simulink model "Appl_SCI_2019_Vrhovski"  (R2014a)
settings: Solver=ode45  StartTime=0.0  StopTime=1000  MaxStep=0.01  RelTol=1e-3
undefined symbols (not defined in the file): deg, H, kg, m, M, mm, N, rad, s, X, Y, Z
libraries: sm_lib x389, nesl_utility x69, simulink x7
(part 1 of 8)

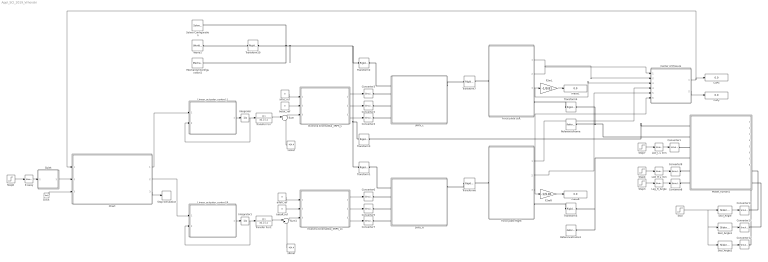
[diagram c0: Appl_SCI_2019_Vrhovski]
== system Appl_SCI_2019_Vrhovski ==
  3RPS_L : Subsystem
  3RPS_R : Subsystem
  Center of Presure : MATLAB Function  TreatAsAtomicUnit=on
  Chart : Stateflow chart  TreatAsAtomicUnit=on
  Clock : Clock
  CoPx : Display
  CoPy : Display
  Converter{1..7,9} (8 alike) : nesl_utility/Simulink-PS Converter  PhysicalDomain=network_engine_domain  SubClassName=ps_input  LeftPortType=input  RightPortType=output  PseudoPeriodic=off  Frequencies=[]  NoiseDistribution=none  NoiseParameters=[]  Unit=mm  AffineConversion=off  InputFiltering=on  SimscapeFilterOrder=2  InputFilterTimeConstant=.01  UdotUserProvided=1
  Converter{8,10..12} (4 alike) : nesl_utility/Simulink-PS Converter  PhysicalDomain=network_engine_domain  SubClassName=ps_input  LeftPortType=input  RightPortType=output  PseudoPeriodic=off  Frequencies=[]  NoiseDistribution=none  NoiseParameters=[]  Unit=rad  AffineConversion=off  InputFiltering=on  SimscapeFilterOrder=2  InputFilterTimeConstant=.01  UdotUserProvided=1
  F2mL : Gain  Gain=-1/9.81
  F2mR : Gain  Gain=-1/9.81
  Force plate Left : Subsystem
  Force plate Right : Subsystem
  Integrator : Integrator
  Integrator1 : Integrator
  Inverzna kinematika_3RPS_L : MATLAB Function  TreatAsAtomicUnit=on
  Inverzna kinematika_3RPS_L1 : MATLAB Function  TreatAsAtomicUnit=on
  K sway : simulink/Math Operations/Slider Gain  low=0  gain=0  high=1
  LLD_L u mm : simulink/Math Operations/Slider Gain  low=0  gain=25  high=340
  LLD_R u mm : simulink/Math Operations/Slider Gain  low=0  gain=0  high=100
  Leg_R_Angle : simulink/Math Operations/Slider Gain  low=-1  gain=0  high=30
  Linear_actuator_control_L : MATLAB Function  TreatAsAtomicUnit=on
  Linear_actuator_control_R : MATLAB Function  TreatAsAtomicUnit=on
  MechanismConfiguration1 : sm_lib/Utilities/Mechanism Configuration  UniformGravity=Constant  GravityVector="[0  0 -9.81]"  GravityUnits=m/s^2  LinearizationDelta=0.001  BlockFunction=simmechanics.library.utilities.mechanism_configuration
  Model_human1 : Subsystem
  Quiet : MATLAB Function  TreatAsAtomicUnit=on
  ReferenceFrame : sm_lib/Frames and Transforms/Reference Frame  BlockFunction=simmechanics.library.frames_transforms.reference_frame
  ReferenceFrame1 : sm_lib/Frames and Transforms/Reference Frame  BlockFunction=simmechanics.library.frames_transforms.reference_frame
  Skol : Step  Time=0  SampleTime=0
  Skol_Angle : simulink/Math Operations/Slider Gain  low=-1  gain=-0.192  high=1
  Skol_Angle1 : simulink/Math Operations/Slider Gain  low=-2  gain=0.078199  high=1
  Skol_Angle2 : simulink/Math Operations/Slider Gain  low=-1  gain=0.09701  high=1
  Solver Configuration : nesl_utility/Solver Configuration  PhysicalDomain=network_engine_domain  SubClassName=solver  LeftPortType=input  RightPortType=generic  Accelerate=off  Tones=[]  Harmonics=[]  SimulateNoise=off  Profile=off  UseLocalSampling=off  EnableSwitchedLinearOptims=on  FrequencyDomain=off  UseCCode=off  RelTol=0.001  AbsTol=1e-06  MinStep=1e-09  ToWorkspace=off  DoDC=off  ResidualTolerance=1e-06  UseLocalSolver=off  LocalSolverChoice=NE_BACKWARD_EULER_ADVANCER  LocalSolverSampleTime=0.001  DoFixedCost=off  MaxNonlinIter=3  MaxModeIter=2  LinearAlgebra=Sparse  DelaysMemoryBudget=1024  AutomaticFiltering=on  FilteringTimeConstant=0.001
  Step3 : Step  Time=0  After=-1  SampleTime=0
  Step4 : Step  Time=0  SampleTime=0
  Step6 : Step  Time=0  SampleTime=0
  Step7 : Step  Time=0  SampleTime=0
  Stop Simulation : Stop
  Sum : Sum  Inputs=|++
  Sum1 : Sum  Inputs=|++
  Transfer Fcn : TransferFcn  Denominator=[0.3 1]
  Transfer Fcn1 : TransferFcn  Denominator=[0.3 1]
  Transform1 : sm_lib/Frames and Transforms/Rigid Transform  TranslationMethod=Cartesian  TranslationLengthUnit=mm  TranslationStandardAxis=+Z  TranslationStandardOffset=0  TranslationCartesianOffset=[0 265 2.5]  TranslationROffset=0  TranslationROffsetUnits=m  TranslationZOffset=0  TranslationZOffsetUnits=m  TranslationThetaOffset=0  TranslationThetaOffsetUnits=deg  RotationMethod=None  RotationAngleUnits=rad  RotationStandardAxis=+Z  RotationAngle=0.66591007177581396  RotationArbitraryAxis=[0.82933268280998906 0.55820538845577061 0.024779941931496435]  FollAlignAxisA=+X  BaseAlignAxisA=+Y  FollAlignAxisB=+Y  BaseAlignAxisB=+Z  BlockFunction=simmechanics.library.frames_transforms.rigid_transform
  Transform10 : sm_lib/Frames and Transforms/Rigid Transform  TranslationMethod=None  TranslationLengthUnit=mm  TranslationStandardAxis=+Z  TranslationStandardOffset=2.5  TranslationCartesianOffset=[0 0 0]  TranslationROffset=0  TranslationROffsetUnits=m  TranslationZOffset=0  TranslationZOffsetUnits=m  TranslationThetaOffset=0  TranslationThetaOffsetUnits=deg  RotationMethod=StandardAxis  RotationAngleUnits=rad  RotationStandardAxis=-Z  RotationAngle=pi/2  RotationArbitraryAxis=[0.82933268280998906 0.55820538845577061 0.024779941931496435]  FollAlignAxisA=+X  BaseAlignAxisA=+Y  FollAlignAxisB=+Y  BaseAlignAxisB=+Z  BlockFunction=simmechanics.library.frames_transforms.rigid_transform
  Transform2 : sm_lib/Frames and Transforms/Rigid Transform  TranslationMethod=Cartesian  TranslationLengthUnit=mm  TranslationStandardAxis=+Z  TranslationStandardOffset=2.5  TranslationCartesianOffset=[0 0 2.5]  TranslationROffset=0  TranslationROffsetUnits=m  TranslationZOffset=0  TranslationZOffsetUnits=m  TranslationThetaOffset=0  TranslationThetaOffsetUnits=deg  RotationMethod=None  RotationAngleUnits=rad  RotationStandardAxis=+Z  RotationAngle=0.66591007177581396  RotationArbitraryAxis=[0.82933268280998906 0.55820538845577061 0.024779941931496435]  FollAlignAxisA=+X  BaseAlignAxisA=+Y  FollAlignAxisB=+Y  BaseAlignAxisB=+Z  BlockFunction=simmechanics.library.frames_transforms.rigid_transform
  Transform3 : sm_lib/Frames and Transforms/Rigid Transform  TranslationMethod=Cartesian  TranslationLengthUnit=mm  TranslationStandardAxis=+Z  TranslationStandardOffset=2.5  TranslationCartesianOffset=[0 265/2 2.5]  TranslationROffset=0  TranslationROffsetUnits=m  TranslationZOffset=0  TranslationZOffsetUnits=m  TranslationThetaOffset=0  TranslationThetaOffsetUnits=deg  RotationMethod=None  RotationAngleUnits=rad  RotationStandardAxis=+Z  RotationAngle=0.66591007177581396  RotationArbitraryAxis=[0.82933268280998906 0.55820538845577061 0.024779941931496435]  FollAlignAxisA=+X  BaseAlignAxisA=+Y  FollAlignAxisB=+Y  BaseAlignAxisB=+Z  BlockFunction=simmechanics.library.frames_transforms.rigid_transform
  Transform4 : sm_lib/Frames and Transforms/Rigid Transform  TranslationMethod=Cartesian  TranslationLengthUnit=mm  TranslationStandardAxis=+Z  TranslationStandardOffset=15  TranslationCartesianOffset=[ 0 0 20]  TranslationROffset=0  TranslationROffsetUnits=m  TranslationZOffset=0  TranslationZOffsetUnits=m  TranslationThetaOffset=0  TranslationThetaOffsetUnits=deg  RotationMethod=None  RotationAngleUnits=rad  RotationStandardAxis=+Z  RotationAngle=2.0943951023931953  RotationArbitraryAxis=[-0.57735026918962584 -0.57735026918962584 -0.57735026918962584]  FollAlignAxisA=+X  BaseAlignAxisA=+Y  FollAlignAxisB=+Y  BaseAlignAxisB=+Z  BlockFunction=simmechanics.library.frames_transforms.rigid_transform
  Transform5 : sm_lib/Frames and Transforms/Rigid Transform  TranslationMethod=Cartesian  TranslationLengthUnit=mm  TranslationStandardAxis=+Z  TranslationStandardOffset=15  TranslationCartesianOffset=[ 0 0 20]  TranslationROffset=0  TranslationROffsetUnits=m  TranslationZOffset=0  TranslationZOffsetUnits=m  TranslationThetaOffset=0  TranslationThetaOffsetUnits=deg  RotationMethod=None  RotationAngleUnits=rad  RotationStandardAxis=+Z  RotationAngle=2.0943951023931953  RotationArbitraryAxis=[-0.57735026918962584 -0.57735026918962584 -0.57735026918962584]  FollAlignAxisA=+X  BaseAlignAxisA=+Y  FollAlignAxisB=+Y  BaseAlignAxisB=+Z  BlockFunction=simmechanics.library.frames_transforms.rigid_transform
  Transform6 : sm_lib/Frames and Transforms/Rigid Transform  TranslationMethod=None  TranslationLengthUnit=mm  TranslationStandardAxis=+Z  TranslationStandardOffset=54.83  TranslationCartesianOffset=[-120 50 70]  TranslationROffset=0  TranslationROffsetUnits=m  TranslationZOffset=0  TranslationZOffsetUnits=m  TranslationThetaOffset=0  TranslationThetaOffsetUnits=deg  RotationMethod=StandardAxis  RotationAngleUnits=rad  RotationStandardAxis=+Z  RotationAngle=pi/2  RotationArbitraryAxis=[0 0 0]  FollAlignAxisA=+X  BaseAlignAxisA=+Y  FollAlignAxisB=+Y  BaseAlignAxisB=+Z  BlockFunction=simmechanics.library.frames_transforms.rigid_transform
  Transform7 : sm_lib/Frames and Transforms/Rigid Transform  TranslationMethod=None  TranslationLengthUnit=mm  TranslationStandardAxis=+Z  TranslationStandardOffset=54.83  TranslationCartesianOffset=[-120 50 70]  TranslationROffset=0  TranslationROffsetUnits=m  TranslationZOffset=0  TranslationZOffsetUnits=m  TranslationThetaOffset=0  TranslationThetaOffsetUnits=deg  RotationMethod=StandardAxis  RotationAngleUnits=rad  RotationStandardAxis=+Z  RotationAngle=pi/2  RotationArbitraryAxis=[0 0 0]  FollAlignAxisA=+X  BaseAlignAxisA=+Y  FollAlignAxisB=+Y  BaseAlignAxisB=+Z  BlockFunction=simmechanics.library.frames_transforms.rigid_transform
  World1 : sm_lib/Frames and Transforms/World Frame  BlockFunction=simmechanics.library.frames_transforms.world_frame
  alfaL_ref : Constant  Value=0
  alfaR_ref : Constant  Value=0
  betaL_ref : Constant  Value=0
  betaR_ref : Constant  Value=0
  masaL : Display
  masaR : Display
  zL0ref : Constant  Value=424.4
  zR0ref : Constant  Value=424.4
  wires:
  Force plate Left/1(CoP_x) -> Center of Presure/1(CoPxL)
  Force plate Left/2(CoP_y) -> Center of Presure/2(CoPyL)
  Force plate Right/1(CoP_x) -> Center of Presure/4(CoPxR)
  Force plate Right/2(CoP_y) -> Center of Presure/5(CoPyR)
  Step7/1 -> LLD_L u mm/1
  LLD_L u mm/1 -> Converter1/1
  Step3/1 -> Leg_R_Angle/1
  Step4/1 -> LLD_R u mm/1
  LLD_R u mm/1 -> Converter9/1
  Force plate Right/3(Fz) -> F2mR/1, Center of Presure/6(FzR)
  F2mL/1 -> masaL/1
  F2mR/1 -> masaR/1
  Force plate Left/3(Fz) -> F2mL/1, Center of Presure/3(FzL)
  Center of Presure/2(CoP_y) -> CoPy/1
  Leg_R_Angle/1 -> Converter8/1
  Inverzna kinematika_3RPS_L/1(d1) -> Converter3/1
  Inverzna kinematika_3RPS_L/2(d2) -> Converter2/1
  Inverzna kinematika_3RPS_L/3(d3) -> Converter4/1
  Inverzna kinematika_3RPS_L1/1(d1) -> Converter6/1
  Inverzna kinematika_3RPS_L1/2(d2) -> Converter5/1
  Inverzna kinematika_3RPS_L1/3(d3) -> Converter7/1
  Center of Presure/1(CoP_x) -> Chart/1(CoM_x), CoPx/1
  alfaL_ref/1 -> Inverzna kinematika_3RPS_L/1(alfa)
  betaL_ref/1 -> Inverzna kinematika_3RPS_L/2(beta)
  alfaR_ref/1 -> Inverzna kinematika_3RPS_L1/1(alfa)
  betaR_ref/1 -> Inverzna kinematika_3RPS_L1/2(beta)
  zL0ref/1 -> Sum/2
  Transfer Fcn1/1 -> Sum1/1
  Sum1/1 -> Inverzna kinematika_3RPS_L1/3(z)
  zR0ref/1 -> Sum1/2
  Skol/1 -> Skol_Angle2/1, Skol_Angle1/1, Skol_Angle/1
  Linear_actuator_control_L/1(u_R) -> Integrator/1
  Integrator/1 -> Linear_actuator_control_L/2(delta_z), Transfer Fcn/1
  Transfer Fcn/1 -> Sum/1
  Linear_actuator_control_R/1(u_R) -> Integrator1/1
  Integrator1/1 -> Transfer Fcn1/1, Linear_actuator_control_R/2(delta_z)
  K sway/1 -> Quiet/1(u)
  Step6/1 -> K sway/1
  Clock/1 -> Chart/3(t)
  Chart/3(end_sim) -> Stop Simulation/1
  Quiet/1(y) -> Chart/2(Q)
  Chart/1(z_ref_L) -> Linear_actuator_control_L/1(delta_z_ref)
  Chart/2(z_ref_R) -> Linear_actuator_control_R/1(delta_z_ref)
  Sum/1 -> Inverzna kinematika_3RPS_L/3(z)
  Skol_Angle2/1 -> Converter12/1
  Skol_Angle1/1 -> Converter11/1
  Skol_Angle/1 -> Converter10/1
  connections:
  3RPS_L/LConn1 -- Transform2/RConn1
  3RPS_L/RConn1 -- Transform7/LConn1
  3RPS_R/LConn1 -- Transform1/RConn1
  Transform6/LConn1 -- 3RPS_R/RConn1
  Transform4/RConn1 -- Model_human1/LConn2 -- ReferenceFrame/RConn1
  Transform5/RConn1 -- Model_human1/LConn4 -- ReferenceFrame1/RConn1
  Model_human1/LConn5 -- Converter9/RConn1
  Transform4/LConn1 -- Force plate Left/RConn1
  Transform5/LConn1 -- Force plate Right/RConn1
  Model_human1/LConn3 -- Converter1/RConn1
  Model_human1/LConn6 -- Converter8/RConn1
  Transform10/RConn1 -- Solver Configuration/RConn1 -- MechanismConfiguration1/RConn1 -- Transform1/LConn1 -- Transform3/LConn1 -- Transform2/LConn1
  Transform7/RConn1 -- Force plate Left/LConn1
  Transform6/RConn1 -- Force plate Right/LConn1
  Transform10/LConn1 -- World1/RConn1
  3RPS_R/LConn4 -- Converter7/RConn1
  3RPS_R/LConn3 -- Converter5/RConn1
  3RPS_R/LConn2 -- Converter6/RConn1
  3RPS_L/LConn2 -- Converter3/RConn1
  3RPS_L/LConn3 -- Converter2/RConn1
  3RPS_L/LConn4 -- Converter4/RConn1
  Transform3/RConn1 -- Model_human1/LConn1
  Model_human1/RConn1 -- Converter10/RConn1
  Model_human1/RConn3 -- Converter11/RConn1
  Converter12/RConn1 -- Model_human1/RConn2

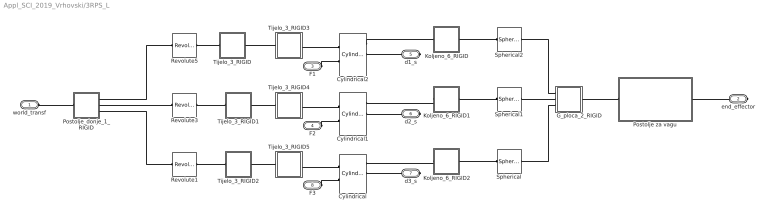
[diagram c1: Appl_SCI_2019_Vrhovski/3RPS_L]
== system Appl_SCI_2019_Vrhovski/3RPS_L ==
  Cylindrical : sm_lib/Joints/Cylindrical Joint  SenseConstraintForce=off  SenseConstraintForceX=off  SenseConstraintForceY=off  SenseConstraintForceZ=off  SenseConstraintTorque=off  SenseConstraintTorqueX=off  SenseConstraintTorqueY=off  SenseConstraintTorqueZ=off  SenseTotalForce=off  SenseTotalForceX=off  SenseTotalForceY=off  SenseTotalForceZ=off  SenseTotalTorque=off  SenseTotalTorqueX=off  SenseTotalTorqueY=off  SenseTotalTorqueZ=off  CompositeWrenchDir=FollowerOnBase  CompositeWrenchFrame=BaseFrame  PzEquilibriumPosition=0  PzEquilibriumPositionUnits=m  PzSpringStiffness=0  PzSpringStiffnessUnits=N/m  PzDampingCoefficient=0  PzDampingCoefficientUnits=s*N/m  PzTorqueActuationMode=ComputedTorque  PzMotionActuationMode=InputMotion  PzSensePosition=on  PzSenseVelocity=on  PzSenseAcceleration=off  PzSenseTorqueForce=off  PzPositionTargetValue=0  PzPositionTargetValueUnits=mm  PzPositionTargetSpecify=on  PzPositionTargetPriority=Low  PzVelocityTargetValue=0  PzVelocityTargetValueUnits=m/s  PzVelocityTargetSpecify=off  PzVelocityTargetPriority=High  RzEquilibriumPosition=0  RzEquilibriumPositionUnits=rad  RzSpringStiffness=0  RzSpringStiffnessUnits=m*N/rad  RzDampingCoefficient=0  RzDampingCoefficientUnits=m*s*N/rad  RzTorqueActuationMode=NoTorque  RzMotionActuationMode=ComputedMotion  RzSensePosition=off  RzSenseVelocity=off  RzSenseAcceleration=off  RzSenseTorqueForce=off  RzPositionTargetValue=149.99999999999969  RzPositionTargetValueUnits=deg  RzPositionTargetSpecify=on  RzPositionTargetPriority=Low  RzVelocityTargetValue=0  RzVelocityTargetValueUnits=deg/s  RzVelocityTargetSpecify=off  RzVelocityTargetPriority=High  BlockFunction=simmechanics.library.joints.cylindrical_joint
  Cylindrical1 : sm_lib/Joints/Cylindrical Joint  SenseConstraintForce=off  SenseConstraintForceX=off  SenseConstraintForceY=off  SenseConstraintForceZ=off  SenseConstraintTorque=off  SenseConstraintTorqueX=off  SenseConstraintTorqueY=off  SenseConstraintTorqueZ=off  SenseTotalForce=off  SenseTotalForceX=off  SenseTotalForceY=off  SenseTotalForceZ=off  SenseTotalTorque=off  SenseTotalTorqueX=off  SenseTotalTorqueY=off  SenseTotalTorqueZ=off  CompositeWrenchDir=FollowerOnBase  CompositeWrenchFrame=BaseFrame  PzEquilibriumPosition=0  PzEquilibriumPositionUnits=m  PzSpringStiffness=0  PzSpringStiffnessUnits=N/m  PzDampingCoefficient=0  PzDampingCoefficientUnits=s*N/m  PzTorqueActuationMode=ComputedTorque  PzMotionActuationMode=InputMotion  PzSensePosition=on  PzSenseVelocity=on  PzSenseAcceleration=off  PzSenseTorqueForce=off  PzPositionTargetValue=0  PzPositionTargetValueUnits=mm  PzPositionTargetSpecify=on  PzPositionTargetPriority=High  PzVelocityTargetValue=0  PzVelocityTargetValueUnits=m/s  PzVelocityTargetSpecify=off  PzVelocityTargetPriority=High  RzEquilibriumPosition=0  RzEquilibriumPositionUnits=rad  RzSpringStiffness=0  RzSpringStiffnessUnits=m*N/rad  RzDampingCoefficient=0  RzDampingCoefficientUnits=m*s*N/rad  RzTorqueActuationMode=NoTorque  RzMotionActuationMode=ComputedMotion  RzSensePosition=off  RzSenseVelocity=off  RzSenseAcceleration=off  RzSenseTorqueForce=off  RzPositionTargetValue=1.1114762716872906  RzPositionTargetValueUnits=deg  RzPositionTargetSpecify=on  RzPositionTargetPriority=Low  RzVelocityTargetValue=0  RzVelocityTargetValueUnits=deg/s  RzVelocityTargetSpecify=off  RzVelocityTargetPriority=High  BlockFunction=simmechanics.library.joints.cylindrical_joint
  Cylindrical2 : sm_lib/Joints/Cylindrical Joint  SenseConstraintForce=off  SenseConstraintForceX=off  SenseConstraintForceY=off  SenseConstraintForceZ=off  SenseConstraintTorque=off  SenseConstraintTorqueX=off  SenseConstraintTorqueY=off  SenseConstraintTorqueZ=off  SenseTotalForce=off  SenseTotalForceX=off  SenseTotalForceY=off  SenseTotalForceZ=off  SenseTotalTorque=off  SenseTotalTorqueX=off  SenseTotalTorqueY=off  SenseTotalTorqueZ=off  CompositeWrenchDir=FollowerOnBase  CompositeWrenchFrame=BaseFrame  PzEquilibriumPosition=0  PzEquilibriumPositionUnits=m  PzSpringStiffness=0  PzSpringStiffnessUnits=N/m  PzDampingCoefficient=0  PzDampingCoefficientUnits=s*N/m  PzTorqueActuationMode=ComputedTorque  PzMotionActuationMode=InputMotion  PzSensePosition=on  PzSenseVelocity=on  PzSenseAcceleration=off  PzSenseTorqueForce=off  PzPositionTargetValue=0  PzPositionTargetValueUnits=mm  PzPositionTargetSpecify=on  PzPositionTargetPriority=High  PzVelocityTargetValue=0  PzVelocityTargetValueUnits=m/s  PzVelocityTargetSpecify=off  PzVelocityTargetPriority=High  RzEquilibriumPosition=0  RzEquilibriumPositionUnits=rad  RzSpringStiffness=0  RzSpringStiffnessUnits=m*N/rad  RzDampingCoefficient=0  RzDampingCoefficientUnits=m*s*N/rad  RzTorqueActuationMode=NoTorque  RzMotionActuationMode=ComputedMotion  RzSensePosition=off  RzSenseVelocity=off  RzSenseAcceleration=off  RzSenseTorqueForce=off  RzPositionTargetValue=-128.14822527507599  RzPositionTargetValueUnits=deg  RzPositionTargetSpecify=on  RzPositionTargetPriority=Low  RzVelocityTargetValue=0  RzVelocityTargetValueUnits=deg/s  RzVelocityTargetSpecify=off  RzVelocityTargetPriority=High  BlockFunction=simmechanics.library.joints.cylindrical_joint
  G_ploca_2_RIGID : Subsystem
  Koljeno_6_RIGID : Subsystem
  Koljeno_6_RIGID1 : Subsystem
  Koljeno_6_RIGID2 : Subsystem
  Postolje za vagu : Subsystem
  Postolje_donje_1_RIGID : Subsystem
  Revolute1 : sm_lib/Joints/Revolute Joint  SenseConstraintForce=off  SenseConstraintForceX=off  SenseConstraintForceY=off  SenseConstraintForceZ=off  SenseConstraintTorque=off  SenseConstraintTorqueX=off  SenseConstraintTorqueY=off  SenseConstraintTorqueZ=off  SenseTotalForce=off  SenseTotalForceX=off  SenseTotalForceY=off  SenseTotalForceZ=off  SenseTotalTorque=off  SenseTotalTorqueX=off  SenseTotalTorqueY=off  SenseTotalTorqueZ=off  CompositeWrenchDir=FollowerOnBase  CompositeWrenchFrame=BaseFrame  EquilibriumPosition=0  EquilibriumPositionUnits=rad  SpringStiffness=0  SpringStiffnessUnits=m*N/rad  DampingCoefficient=0  DampingCoefficientUnits=m*s*N/rad  TorqueActuationMode=NoTorque  MotionActuationMode=ComputedMotion  SensePosition=off  SenseVelocity=off  SenseAcceleration=off  SenseTorqueForce=off  PositionTargetValue=-169.15902616998602  PositionTargetValueUnits=deg  PositionTargetSpecify=on  PositionTargetPriority=Low  VelocityTargetValue=0  VelocityTargetValueUnits=deg/s  VelocityTargetSpecify=off  VelocityTargetPriority=High  BlockFunction=simmechanics.library.joints.revolute_joint
  Revolute3 : sm_lib/Joints/Revolute Joint  SenseConstraintForce=off  SenseConstraintForceX=off  SenseConstraintForceY=off  SenseConstraintForceZ=off  SenseConstraintTorque=off  SenseConstraintTorqueX=off  SenseConstraintTorqueY=off  SenseConstraintTorqueZ=off  SenseTotalForce=off  SenseTotalForceX=off  SenseTotalForceY=off  SenseTotalForceZ=off  SenseTotalTorque=off  SenseTotalTorqueX=off  SenseTotalTorqueY=off  SenseTotalTorqueZ=off  CompositeWrenchDir=FollowerOnBase  CompositeWrenchFrame=BaseFrame  EquilibriumPosition=0  EquilibriumPositionUnits=rad  SpringStiffness=0  SpringStiffnessUnits=m*N/rad  DampingCoefficient=0  DampingCoefficientUnits=m*s*N/rad  TorqueActuationMode=NoTorque  MotionActuationMode=ComputedMotion  SensePosition=off  SenseVelocity=off  SenseAcceleration=off  SenseTorqueForce=off  PositionTargetValue=169.15902616998767  PositionTargetValueUnits=deg  PositionTargetSpecify=on  PositionTargetPriority=Low  VelocityTargetValue=0  VelocityTargetValueUnits=deg/s  VelocityTargetSpecify=off  VelocityTargetPriority=High  BlockFunction=simmechanics.library.joints.revolute_joint
  Revolute5 : sm_lib/Joints/Revolute Joint  SenseConstraintForce=off  SenseConstraintForceX=off  SenseConstraintForceY=off  SenseConstraintForceZ=off  SenseConstraintTorque=off  SenseConstraintTorqueX=off  SenseConstraintTorqueY=off  SenseConstraintTorqueZ=off  SenseTotalForce=off  SenseTotalForceX=off  SenseTotalForceY=off  SenseTotalForceZ=off  SenseTotalTorque=off  SenseTotalTorqueX=off  SenseTotalTorqueY=off  SenseTotalTorqueZ=off  CompositeWrenchDir=FollowerOnBase  CompositeWrenchFrame=BaseFrame  EquilibriumPosition=0  EquilibriumPositionUnits=rad  SpringStiffness=0  SpringStiffnessUnits=m*N/rad  DampingCoefficient=0  DampingCoefficientUnits=m*s*N/rad  TorqueActuationMode=NoTorque  MotionActuationMode=ComputedMotion  SensePosition=off  SenseVelocity=off  SenseAcceleration=off  SenseTorqueForce=off  PositionTargetValue=79.159026169986646  PositionTargetValueUnits=deg  PositionTargetSpecify=on  PositionTargetPriority=Low  VelocityTargetValue=0  VelocityTargetValueUnits=deg/s  VelocityTargetSpecify=off  VelocityTargetPriority=High  BlockFunction=simmechanics.library.joints.revolute_joint
  Spherical : sm_lib/Joints/Spherical Joint  SenseConstraintForce=off  SenseConstraintForceX=off  SenseConstraintForceY=off  SenseConstraintForceZ=off  SenseConstraintTorque=off  SenseConstraintTorqueX=off  SenseConstraintTorqueY=off  SenseConstraintTorqueZ=off  SenseTotalForce=off  SenseTotalForceX=off  SenseTotalForceY=off  SenseTotalForceZ=off  SenseTotalTorque=off  SenseTotalTorqueX=off  SenseTotalTorqueY=off  SenseTotalTorqueZ=off  CompositeWrenchDir=FollowerOnBase  CompositeWrenchFrame=BaseFrame  DefPosRotationMethod=None  DefPosRotationAngleUnits=deg  DefPosRotationStandardAxis=+Z  DefPosRotationAngle=0  DefPosRotationArbitraryAxis=[0 0 1]  DefPosFollAlignAxisA=+X  DefPosBaseAlignAxisA=+Y  DefPosFollAlignAxisB=+Y  DefPosBaseAlignAxisB=+Z  EqPosRotationMethod=None  EqPosRotationAngleUnits=deg  EqPosRotationStandardAxis=+Z  EqPosRotationAngle=0  EqPosRotationArbitraryAxis=[0 0 1]  EqPosFollAlignAxisA=+X  EqPosBaseAlignAxisA=+Y  EqPosFollAlignAxisB=+Y  EqPosBaseAlignAxisB=+Z  SpringStiffness=0  SpringStiffnessUnits=m*N/rad  DampingCoefficient=0  DampingCoefficientUnits=m*s*N/rad  ActuateTorqueX=off  ActuateTorqueY=off  ActuateTorqueZ=off  ActuateTorque=off  TorqueActuationMode=NoTorque  MotionActuationMode=ComputedMotion  ActuationFrame=BaseFrame  SensePosition=off  SenseVelocityX=off  SenseVelocityY=off  SenseVelocityZ=off  SenseVelocity=off  SenseAccelerationX=off  SenseAccelerationY=off  SenseAccelerationZ=off  SenseAcceleration=off  SenseTorqueX=off  SenseTorqueY=off  SenseTorqueZ=off  SenseTorqueForce=off  SensingFrame=FollowerFrame  PositionTargetRotationMethod=ArbitraryAxis  PositionTargetRotationAngleUnits=deg  PositionTargetRotationStandardAxis=+Z  PositionTargetRotationAngle=99.696739951188775  PositionTargetRotationArbitraryAxis=[-0.99752584719718795 0.068907511443980704 -0.013926199773456341]  PositionTargetFollAlignAxisA=+X  PositionTargetBaseAlignAxisA=+Y  PositionTargetFollAlignAxisB=+Y  PositionTargetBaseAlignAxisB=+Z  PositionTargetSpecify=on  PositionTargetPriority=Low  VelocityTargetValue=[0 0 0]  VelocityTargetValueUnits=deg/s  VelocityTargetSpecify=off  VelocityTargetPriority=High  VelocityTargetInFollowerFrame=on  BlockFunction=simmechanics.library.joints.spherical_joint
  Spherical1 : sm_lib/Joints/Spherical Joint  SenseConstraintForce=off  SenseConstraintForceX=off  SenseConstraintForceY=off  SenseConstraintForceZ=off  SenseConstraintTorque=off  SenseConstraintTorqueX=off  SenseConstraintTorqueY=off  SenseConstraintTorqueZ=off  SenseTotalForce=off  SenseTotalForceX=off  SenseTotalForceY=off  SenseTotalForceZ=off  SenseTotalTorque=off  SenseTotalTorqueX=off  SenseTotalTorqueY=off  SenseTotalTorqueZ=off  CompositeWrenchDir=FollowerOnBase  CompositeWrenchFrame=BaseFrame  DefPosRotationMethod=None  DefPosRotationAngleUnits=deg  DefPosRotationStandardAxis=+Z  DefPosRotationAngle=0  DefPosRotationArbitraryAxis=[0 0 1]  DefPosFollAlignAxisA=+X  DefPosBaseAlignAxisA=+Y  DefPosFollAlignAxisB=+Y  DefPosBaseAlignAxisB=+Z  EqPosRotationMethod=None  EqPosRotationAngleUnits=deg  EqPosRotationStandardAxis=+Z  EqPosRotationAngle=0  EqPosRotationArbitraryAxis=[0 0 1]  EqPosFollAlignAxisA=+X  EqPosBaseAlignAxisA=+Y  EqPosFollAlignAxisB=+Y  EqPosBaseAlignAxisB=+Z  SpringStiffness=0  SpringStiffnessUnits=m*N/rad  DampingCoefficient=0  DampingCoefficientUnits=m*s*N/rad  ActuateTorqueX=off  ActuateTorqueY=off  ActuateTorqueZ=off  ActuateTorque=off  TorqueActuationMode=NoTorque  MotionActuationMode=ComputedMotion  ActuationFrame=BaseFrame  SensePosition=off  SenseVelocityX=off  SenseVelocityY=off  SenseVelocityZ=off  SenseVelocity=off  SenseAccelerationX=off  SenseAccelerationY=off  SenseAccelerationZ=off  SenseAcceleration=off  SenseTorqueX=off  SenseTorqueY=off  SenseTorqueZ=off  SenseTorqueForce=off  SensingFrame=FollowerFrame  PositionTargetRotationMethod=None  PositionTargetRotationAngleUnits=deg  PositionTargetRotationStandardAxis=+Z  PositionTargetRotationAngle=0  PositionTargetRotationArbitraryAxis=[0 0 1]  PositionTargetFollAlignAxisA=+X  PositionTargetBaseAlignAxisA=+Y  PositionTargetFollAlignAxisB=+Y  PositionTargetBaseAlignAxisB=+Z  PositionTargetSpecify=off  PositionTargetPriority=High  VelocityTargetValue=[0 0 0]  VelocityTargetValueUnits=deg/s  VelocityTargetSpecify=off  VelocityTargetPriority=High  VelocityTargetInFollowerFrame=on  BlockFunction=simmechanics.library.joints.spherical_joint
  Spherical2 : sm_lib/Joints/Spherical Joint  SenseConstraintForce=off  SenseConstraintForceX=off  SenseConstraintForceY=off  SenseConstraintForceZ=off  SenseConstraintTorque=off  SenseConstraintTorqueX=off  SenseConstraintTorqueY=off  SenseConstraintTorqueZ=off  SenseTotalForce=off  SenseTotalForceX=off  SenseTotalForceY=off  SenseTotalForceZ=off  SenseTotalTorque=off  SenseTotalTorqueX=off  SenseTotalTorqueY=off  SenseTotalTorqueZ=off  CompositeWrenchDir=FollowerOnBase  CompositeWrenchFrame=BaseFrame  DefPosRotationMethod=None  DefPosRotationAngleUnits=deg  DefPosRotationStandardAxis=+Z  DefPosRotationAngle=0  DefPosRotationArbitraryAxis=[0 0 1]  DefPosFollAlignAxisA=+X  DefPosBaseAlignAxisA=+Y  DefPosFollAlignAxisB=+Y  DefPosBaseAlignAxisB=+Z  EqPosRotationMethod=None  EqPosRotationAngleUnits=deg  EqPosRotationStandardAxis=+Z  EqPosRotationAngle=0  EqPosRotationArbitraryAxis=[0 0 1]  EqPosFollAlignAxisA=+X  EqPosBaseAlignAxisA=+Y  EqPosFollAlignAxisB=+Y  EqPosBaseAlignAxisB=+Z  SpringStiffness=0  SpringStiffnessUnits=m*N/rad  DampingCoefficient=0  DampingCoefficientUnits=m*s*N/rad  ActuateTorqueX=off  ActuateTorqueY=off  ActuateTorqueZ=off  ActuateTorque=off  TorqueActuationMode=NoTorque  MotionActuationMode=ComputedMotion  ActuationFrame=BaseFrame  SensePosition=off  SenseVelocityX=off  SenseVelocityY=off  SenseVelocityZ=off  SenseVelocity=off  SenseAccelerationX=off  SenseAccelerationY=off  SenseAccelerationZ=off  SenseAcceleration=off  SenseTorqueX=off  SenseTorqueY=off  SenseTorqueZ=off  SenseTorqueForce=off  SensingFrame=FollowerFrame  PositionTargetRotationMethod=None  PositionTargetRotationAngleUnits=deg  PositionTargetRotationStandardAxis=+Z  PositionTargetRotationAngle=0  PositionTargetRotationArbitraryAxis=[0 0 1]  PositionTargetFollAlignAxisA=+X  PositionTargetBaseAlignAxisA=+Y  PositionTargetFollAlignAxisB=+Y  PositionTargetBaseAlignAxisB=+Z  PositionTargetSpecify=off  PositionTargetPriority=High  VelocityTargetValue=[0 0 0]  VelocityTargetValueUnits=deg/s  VelocityTargetSpecify=off  VelocityTargetPriority=High  VelocityTargetInFollowerFrame=on  BlockFunction=simmechanics.library.joints.spherical_joint
  Tijelo_3_RIGID : Subsystem
  Tijelo_3_RIGID1 : Subsystem
  Tijelo_3_RIGID2 : Subsystem
  Tijelo_3_RIGID3 : Subsystem
  Tijelo_3_RIGID4 : Subsystem
  Tijelo_3_RIGID5 : Subsystem
  world_transf : PMIOPort  Port=1  Side=Left
  end_effector : PMIOPort  Port=2  Side=Right
  F1 : PMIOPort  Port=3  Side=Left
  F2 : PMIOPort  Port=4  Side=Left
  d1_s : PMIOPort  Port=5  Side=Right
  d2_s : PMIOPort  Port=6  Side=Right
  d3_s : PMIOPort  Port=7  Side=Right
  F3 : PMIOPort  Port=8  Side=Left
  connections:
  Postolje_donje_1_RIGID/RConn3 -- Revolute1/LConn1
  Koljeno_6_RIGID2/RConn1 -- Spherical/LConn1
  Koljeno_6_RIGID1/RConn1 -- Spherical1/LConn1
  G_ploca_2_RIGID/LConn2 -- Spherical1/RConn1
  G_ploca_2_RIGID/LConn1 -- Spherical2/RConn1
  G_ploca_2_RIGID/LConn3 -- Spherical/RConn1
  Revolute5/RConn1 -- Tijelo_3_RIGID/LConn1
  Koljeno_6_RIGID/RConn1 -- Spherical2/LConn1
  Postolje_donje_1_RIGID/RConn1 -- Revolute5/LConn1
  Tijelo_3_RIGID2/LConn1 -- Revolute1/RConn1
  Postolje_donje_1_RIGID/RConn2 -- Revolute3/LConn1
  d2_s/RConn1 -- Cylindrical1/RConn2
  d3_s/RConn1 -- Cylindrical/RConn2
  Cylindrical2/RConn1 -- Koljeno_6_RIGID/LConn1
  F3/RConn1 -- Cylindrical/LConn2
  d1_s/RConn1 -- Cylindrical2/RConn2
  Tijelo_3_RIGID1/LConn1 -- Revolute3/RConn1
  F1/RConn1 -- Cylindrical2/LConn2
  Koljeno_6_RIGID1/LConn1 -- Cylindrical1/RConn1
  F2/RConn1 -- Cylindrical1/LConn2
  Koljeno_6_RIGID2/LConn1 -- Cylindrical/RConn1
  world_transf/RConn1 -- Postolje_donje_1_RIGID/LConn1
  G_ploca_2_RIGID/RConn1 -- Postolje za vagu/LConn1
  Postolje za vagu/RConn1 -- end_effector/RConn1
  Tijelo_3_RIGID/RConn1 -- Tijelo_3_RIGID3/LConn1
  Tijelo_3_RIGID3/RConn1 -- Cylindrical2/LConn1
  Tijelo_3_RIGID1/RConn1 -- Tijelo_3_RIGID4/LConn1
  Tijelo_3_RIGID4/RConn1 -- Cylindrical1/LConn1
  Tijelo_3_RIGID2/RConn1 -- Tijelo_3_RIGID5/LConn1
  Tijelo_3_RIGID5/RConn1 -- Cylindrical/LConn1

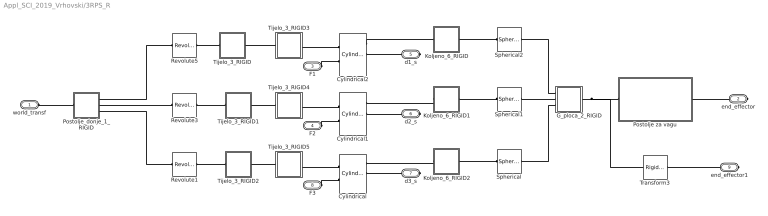
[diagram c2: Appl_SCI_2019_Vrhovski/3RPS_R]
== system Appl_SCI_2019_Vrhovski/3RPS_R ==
  Cylindrical : sm_lib/Joints/Cylindrical Joint  SenseConstraintForce=off  SenseConstraintForceX=off  SenseConstraintForceY=off  SenseConstraintForceZ=off  SenseConstraintTorque=off  SenseConstraintTorqueX=off  SenseConstraintTorqueY=off  SenseConstraintTorqueZ=off  SenseTotalForce=off  SenseTotalForceX=off  SenseTotalForceY=off  SenseTotalForceZ=off  SenseTotalTorque=off  SenseTotalTorqueX=off  SenseTotalTorqueY=off  SenseTotalTorqueZ=off  CompositeWrenchDir=FollowerOnBase  CompositeWrenchFrame=BaseFrame  PzEquilibriumPosition=0  PzEquilibriumPositionUnits=m  PzSpringStiffness=0  PzSpringStiffnessUnits=N/m  PzDampingCoefficient=0  PzDampingCoefficientUnits=s*N/m  PzTorqueActuationMode=ComputedTorque  PzMotionActuationMode=InputMotion  PzSensePosition=on  PzSenseVelocity=on  PzSenseAcceleration=off  PzSenseTorqueForce=off  PzPositionTargetValue=0  PzPositionTargetValueUnits=mm  PzPositionTargetSpecify=on  PzPositionTargetPriority=Low  PzVelocityTargetValue=0  PzVelocityTargetValueUnits=m/s  PzVelocityTargetSpecify=off  PzVelocityTargetPriority=High  RzEquilibriumPosition=0  RzEquilibriumPositionUnits=rad  RzSpringStiffness=0  RzSpringStiffnessUnits=m*N/rad  RzDampingCoefficient=0  RzDampingCoefficientUnits=m*s*N/rad  RzTorqueActuationMode=NoTorque  RzMotionActuationMode=ComputedMotion  RzSensePosition=off  RzSenseVelocity=off  RzSenseAcceleration=off  RzSenseTorqueForce=off  RzPositionTargetValue=149.99999999999969  RzPositionTargetValueUnits=deg  RzPositionTargetSpecify=on  RzPositionTargetPriority=Low  RzVelocityTargetValue=0  RzVelocityTargetValueUnits=deg/s  RzVelocityTargetSpecify=off  RzVelocityTargetPriority=High  BlockFunction=simmechanics.library.joints.cylindrical_joint
  Cylindrical1 : sm_lib/Joints/Cylindrical Joint  SenseConstraintForce=off  SenseConstraintForceX=off  SenseConstraintForceY=off  SenseConstraintForceZ=off  SenseConstraintTorque=off  SenseConstraintTorqueX=off  SenseConstraintTorqueY=off  SenseConstraintTorqueZ=off  SenseTotalForce=off  SenseTotalForceX=off  SenseTotalForceY=off  SenseTotalForceZ=off  SenseTotalTorque=off  SenseTotalTorqueX=off  SenseTotalTorqueY=off  SenseTotalTorqueZ=off  CompositeWrenchDir=FollowerOnBase  CompositeWrenchFrame=BaseFrame  PzEquilibriumPosition=0  PzEquilibriumPositionUnits=m  PzSpringStiffness=0  PzSpringStiffnessUnits=N/m  PzDampingCoefficient=0  PzDampingCoefficientUnits=s*N/m  PzTorqueActuationMode=ComputedTorque  PzMotionActuationMode=InputMotion  PzSensePosition=on  PzSenseVelocity=on  PzSenseAcceleration=off  PzSenseTorqueForce=off  PzPositionTargetValue=0  PzPositionTargetValueUnits=mm  PzPositionTargetSpecify=on  PzPositionTargetPriority=High  PzVelocityTargetValue=0  PzVelocityTargetValueUnits=m/s  PzVelocityTargetSpecify=off  PzVelocityTargetPriority=High  RzEquilibriumPosition=0  RzEquilibriumPositionUnits=rad  RzSpringStiffness=0  RzSpringStiffnessUnits=m*N/rad  RzDampingCoefficient=0  RzDampingCoefficientUnits=m*s*N/rad  RzTorqueActuationMode=NoTorque  RzMotionActuationMode=ComputedMotion  RzSensePosition=off  RzSenseVelocity=off  RzSenseAcceleration=off  RzSenseTorqueForce=off  RzPositionTargetValue=1.1114762716872906  RzPositionTargetValueUnits=deg  RzPositionTargetSpecify=on  RzPositionTargetPriority=Low  RzVelocityTargetValue=0  RzVelocityTargetValueUnits=deg/s  RzVelocityTargetSpecify=off  RzVelocityTargetPriority=High  BlockFunction=simmechanics.library.joints.cylindrical_joint
  Cylindrical2 : sm_lib/Joints/Cylindrical Joint  SenseConstraintForce=off  SenseConstraintForceX=off  SenseConstraintForceY=off  SenseConstraintForceZ=off  SenseConstraintTorque=off  SenseConstraintTorqueX=off  SenseConstraintTorqueY=off  SenseConstraintTorqueZ=off  SenseTotalForce=off  SenseTotalForceX=off  SenseTotalForceY=off  SenseTotalForceZ=off  SenseTotalTorque=off  SenseTotalTorqueX=off  SenseTotalTorqueY=off  SenseTotalTorqueZ=off  CompositeWrenchDir=FollowerOnBase  CompositeWrenchFrame=BaseFrame  PzEquilibriumPosition=0  PzEquilibriumPositionUnits=m  PzSpringStiffness=0  PzSpringStiffnessUnits=N/m  PzDampingCoefficient=0  PzDampingCoefficientUnits=s*N/m  PzTorqueActuationMode=ComputedTorque  PzMotionActuationMode=InputMotion  PzSensePosition=on  PzSenseVelocity=on  PzSenseAcceleration=off  PzSenseTorqueForce=off  PzPositionTargetValue=0  PzPositionTargetValueUnits=mm  PzPositionTargetSpecify=on  PzPositionTargetPriority=High  PzVelocityTargetValue=0  PzVelocityTargetValueUnits=m/s  PzVelocityTargetSpecify=off  PzVelocityTargetPriority=High  RzEquilibriumPosition=0  RzEquilibriumPositionUnits=rad  RzSpringStiffness=0  RzSpringStiffnessUnits=m*N/rad  RzDampingCoefficient=0  RzDampingCoefficientUnits=m*s*N/rad  RzTorqueActuationMode=NoTorque  RzMotionActuationMode=ComputedMotion  RzSensePosition=off  RzSenseVelocity=off  RzSenseAcceleration=off  RzSenseTorqueForce=off  RzPositionTargetValue=-128.14822527507599  RzPositionTargetValueUnits=deg  RzPositionTargetSpecify=on  RzPositionTargetPriority=Low  RzVelocityTargetValue=0  RzVelocityTargetValueUnits=deg/s  RzVelocityTargetSpecify=off  RzVelocityTargetPriority=High  BlockFunction=simmechanics.library.joints.cylindrical_joint
  G_ploca_2_RIGID : Subsystem
  Koljeno_6_RIGID : Subsystem
  Koljeno_6_RIGID1 : Subsystem
  Koljeno_6_RIGID2 : Subsystem
  Postolje za vagu : Subsystem
  Postolje_donje_1_RIGID : Subsystem
  Revolute1 : sm_lib/Joints/Revolute Joint  SenseConstraintForce=off  SenseConstraintForceX=off  SenseConstraintForceY=off  SenseConstraintForceZ=off  SenseConstraintTorque=off  SenseConstraintTorqueX=off  SenseConstraintTorqueY=off  SenseConstraintTorqueZ=off  SenseTotalForce=off  SenseTotalForceX=off  SenseTotalForceY=off  SenseTotalForceZ=off  SenseTotalTorque=off  SenseTotalTorqueX=off  SenseTotalTorqueY=off  SenseTotalTorqueZ=off  CompositeWrenchDir=FollowerOnBase  CompositeWrenchFrame=BaseFrame  EquilibriumPosition=0  EquilibriumPositionUnits=rad  SpringStiffness=0  SpringStiffnessUnits=m*N/rad  DampingCoefficient=0  DampingCoefficientUnits=m*s*N/rad  TorqueActuationMode=NoTorque  MotionActuationMode=ComputedMotion  SensePosition=off  SenseVelocity=off  SenseAcceleration=off  SenseTorqueForce=off  PositionTargetValue=-169.15902616998602  PositionTargetValueUnits=deg  PositionTargetSpecify=on  PositionTargetPriority=Low  VelocityTargetValue=0  VelocityTargetValueUnits=deg/s  VelocityTargetSpecify=off  VelocityTargetPriority=High  BlockFunction=simmechanics.library.joints.revolute_joint
  Revolute3 : sm_lib/Joints/Revolute Joint  SenseConstraintForce=off  SenseConstraintForceX=off  SenseConstraintForceY=off  SenseConstraintForceZ=off  SenseConstraintTorque=off  SenseConstraintTorqueX=off  SenseConstraintTorqueY=off  SenseConstraintTorqueZ=off  SenseTotalForce=off  SenseTotalForceX=off  SenseTotalForceY=off  SenseTotalForceZ=off  SenseTotalTorque=off  SenseTotalTorqueX=off  SenseTotalTorqueY=off  SenseTotalTorqueZ=off  CompositeWrenchDir=FollowerOnBase  CompositeWrenchFrame=BaseFrame  EquilibriumPosition=0  EquilibriumPositionUnits=rad  SpringStiffness=0  SpringStiffnessUnits=m*N/rad  DampingCoefficient=0  DampingCoefficientUnits=m*s*N/rad  TorqueActuationMode=NoTorque  MotionActuationMode=ComputedMotion  SensePosition=off  SenseVelocity=off  SenseAcceleration=off  SenseTorqueForce=off  PositionTargetValue=169.15902616998767  PositionTargetValueUnits=deg  PositionTargetSpecify=on  PositionTargetPriority=Low  VelocityTargetValue=0  VelocityTargetValueUnits=deg/s  VelocityTargetSpecify=off  VelocityTargetPriority=High  BlockFunction=simmechanics.library.joints.revolute_joint
  Revolute5 : sm_lib/Joints/Revolute Joint  SenseConstraintForce=off  SenseConstraintForceX=off  SenseConstraintForceY=off  SenseConstraintForceZ=off  SenseConstraintTorque=off  SenseConstraintTorqueX=off  SenseConstraintTorqueY=off  SenseConstraintTorqueZ=off  SenseTotalForce=off  SenseTotalForceX=off  SenseTotalForceY=off  SenseTotalForceZ=off  SenseTotalTorque=off  SenseTotalTorqueX=off  SenseTotalTorqueY=off  SenseTotalTorqueZ=off  CompositeWrenchDir=FollowerOnBase  CompositeWrenchFrame=BaseFrame  EquilibriumPosition=0  EquilibriumPositionUnits=rad  SpringStiffness=0  SpringStiffnessUnits=m*N/rad  DampingCoefficient=0  DampingCoefficientUnits=m*s*N/rad  TorqueActuationMode=NoTorque  MotionActuationMode=ComputedMotion  SensePosition=off  SenseVelocity=off  SenseAcceleration=off  SenseTorqueForce=off  PositionTargetValue=79.159026169986646  PositionTargetValueUnits=deg  PositionTargetSpecify=on  PositionTargetPriority=Low  VelocityTargetValue=0  VelocityTargetValueUnits=deg/s  VelocityTargetSpecify=off  VelocityTargetPriority=High  BlockFunction=simmechanics.library.joints.revolute_joint
  Spherical : sm_lib/Joints/Spherical Joint  SenseConstraintForce=off  SenseConstraintForceX=off  SenseConstraintForceY=off  SenseConstraintForceZ=off  SenseConstraintTorque=off  SenseConstraintTorqueX=off  SenseConstraintTorqueY=off  SenseConstraintTorqueZ=off  SenseTotalForce=off  SenseTotalForceX=off  SenseTotalForceY=off  SenseTotalForceZ=off  SenseTotalTorque=off  SenseTotalTorqueX=off  SenseTotalTorqueY=off  SenseTotalTorqueZ=off  CompositeWrenchDir=FollowerOnBase  CompositeWrenchFrame=BaseFrame  DefPosRotationMethod=None  DefPosRotationAngleUnits=deg  DefPosRotationStandardAxis=+Z  DefPosRotationAngle=0  DefPosRotationArbitraryAxis=[0 0 1]  DefPosFollAlignAxisA=+X  DefPosBaseAlignAxisA=+Y  DefPosFollAlignAxisB=+Y  DefPosBaseAlignAxisB=+Z  EqPosRotationMethod=None  EqPosRotationAngleUnits=deg  EqPosRotationStandardAxis=+Z  EqPosRotationAngle=0  EqPosRotationArbitraryAxis=[0 0 1]  EqPosFollAlignAxisA=+X  EqPosBaseAlignAxisA=+Y  EqPosFollAlignAxisB=+Y  EqPosBaseAlignAxisB=+Z  SpringStiffness=0  SpringStiffnessUnits=m*N/rad  DampingCoefficient=0  DampingCoefficientUnits=m*s*N/rad  ActuateTorqueX=off  ActuateTorqueY=off  ActuateTorqueZ=off  ActuateTorque=off  TorqueActuationMode=NoTorque  MotionActuationMode=ComputedMotion  ActuationFrame=BaseFrame  SensePosition=off  SenseVelocityX=off  SenseVelocityY=off  SenseVelocityZ=off  SenseVelocity=off  SenseAccelerationX=off  SenseAccelerationY=off  SenseAccelerationZ=off  SenseAcceleration=off  SenseTorqueX=off  SenseTorqueY=off  SenseTorqueZ=off  SenseTorqueForce=off  SensingFrame=FollowerFrame  PositionTargetRotationMethod=ArbitraryAxis  PositionTargetRotationAngleUnits=deg  PositionTargetRotationStandardAxis=+Z  PositionTargetRotationAngle=99.696739951188775  PositionTargetRotationArbitraryAxis=[-0.99752584719718795 0.068907511443980704 -0.013926199773456341]  PositionTargetFollAlignAxisA=+X  PositionTargetBaseAlignAxisA=+Y  PositionTargetFollAlignAxisB=+Y  PositionTargetBaseAlignAxisB=+Z  PositionTargetSpecify=on  PositionTargetPriority=Low  VelocityTargetValue=[0 0 0]  VelocityTargetValueUnits=deg/s  VelocityTargetSpecify=off  VelocityTargetPriority=High  VelocityTargetInFollowerFrame=on  BlockFunction=simmechanics.library.joints.spherical_joint
  Spherical1 : sm_lib/Joints/Spherical Joint  SenseConstraintForce=off  SenseConstraintForceX=off  SenseConstraintForceY=off  SenseConstraintForceZ=off  SenseConstraintTorque=off  SenseConstraintTorqueX=off  SenseConstraintTorqueY=off  SenseConstraintTorqueZ=off  SenseTotalForce=off  SenseTotalForceX=off  SenseTotalForceY=off  SenseTotalForceZ=off  SenseTotalTorque=off  SenseTotalTorqueX=off  SenseTotalTorqueY=off  SenseTotalTorqueZ=off  CompositeWrenchDir=FollowerOnBase  CompositeWrenchFrame=BaseFrame  DefPosRotationMethod=None  DefPosRotationAngleUnits=deg  DefPosRotationStandardAxis=+Z  DefPosRotationAngle=0  DefPosRotationArbitraryAxis=[0 0 1]  DefPosFollAlignAxisA=+X  DefPosBaseAlignAxisA=+Y  DefPosFollAlignAxisB=+Y  DefPosBaseAlignAxisB=+Z  EqPosRotationMethod=None  EqPosRotationAngleUnits=deg  EqPosRotationStandardAxis=+Z  EqPosRotationAngle=0  EqPosRotationArbitraryAxis=[0 0 1]  EqPosFollAlignAxisA=+X  EqPosBaseAlignAxisA=+Y  EqPosFollAlignAxisB=+Y  EqPosBaseAlignAxisB=+Z  SpringStiffness=0  SpringStiffnessUnits=m*N/rad  DampingCoefficient=0  DampingCoefficientUnits=m*s*N/rad  ActuateTorqueX=off  ActuateTorqueY=off  ActuateTorqueZ=off  ActuateTorque=off  TorqueActuationMode=NoTorque  MotionActuationMode=ComputedMotion  ActuationFrame=BaseFrame  SensePosition=off  SenseVelocityX=off  SenseVelocityY=off  SenseVelocityZ=off  SenseVelocity=off  SenseAccelerationX=off  SenseAccelerationY=off  SenseAccelerationZ=off  SenseAcceleration=off  SenseTorqueX=off  SenseTorqueY=off  SenseTorqueZ=off  SenseTorqueForce=off  SensingFrame=FollowerFrame  PositionTargetRotationMethod=None  PositionTargetRotationAngleUnits=deg  PositionTargetRotationStandardAxis=+Z  PositionTargetRotationAngle=0  PositionTargetRotationArbitraryAxis=[0 0 1]  PositionTargetFollAlignAxisA=+X  PositionTargetBaseAlignAxisA=+Y  PositionTargetFollAlignAxisB=+Y  PositionTargetBaseAlignAxisB=+Z  PositionTargetSpecify=off  PositionTargetPriority=High  VelocityTargetValue=[0 0 0]  VelocityTargetValueUnits=deg/s  VelocityTargetSpecify=off  VelocityTargetPriority=High  VelocityTargetInFollowerFrame=on  BlockFunction=simmechanics.library.joints.spherical_joint
  Spherical2 : sm_lib/Joints/Spherical Joint  SenseConstraintForce=off  SenseConstraintForceX=off  SenseConstraintForceY=off  SenseConstraintForceZ=off  SenseConstraintTorque=off  SenseConstraintTorqueX=off  SenseConstraintTorqueY=off  SenseConstraintTorqueZ=off  SenseTotalForce=off  SenseTotalForceX=off  SenseTotalForceY=off  SenseTotalForceZ=off  SenseTotalTorque=off  SenseTotalTorqueX=off  SenseTotalTorqueY=off  SenseTotalTorqueZ=off  CompositeWrenchDir=FollowerOnBase  CompositeWrenchFrame=BaseFrame  DefPosRotationMethod=None  DefPosRotationAngleUnits=deg  DefPosRotationStandardAxis=+Z  DefPosRotationAngle=0  DefPosRotationArbitraryAxis=[0 0 1]  DefPosFollAlignAxisA=+X  DefPosBaseAlignAxisA=+Y  DefPosFollAlignAxisB=+Y  DefPosBaseAlignAxisB=+Z  EqPosRotationMethod=None  EqPosRotationAngleUnits=deg  EqPosRotationStandardAxis=+Z  EqPosRotationAngle=0  EqPosRotationArbitraryAxis=[0 0 1]  EqPosFollAlignAxisA=+X  EqPosBaseAlignAxisA=+Y  EqPosFollAlignAxisB=+Y  EqPosBaseAlignAxisB=+Z  SpringStiffness=0  SpringStiffnessUnits=m*N/rad  DampingCoefficient=0  DampingCoefficientUnits=m*s*N/rad  ActuateTorqueX=off  ActuateTorqueY=off  ActuateTorqueZ=off  ActuateTorque=off  TorqueActuationMode=NoTorque  MotionActuationMode=ComputedMotion  ActuationFrame=BaseFrame  SensePosition=off  SenseVelocityX=off  SenseVelocityY=off  SenseVelocityZ=off  SenseVelocity=off  SenseAccelerationX=off  SenseAccelerationY=off  SenseAccelerationZ=off  SenseAcceleration=off  SenseTorqueX=off  SenseTorqueY=off  SenseTorqueZ=off  SenseTorqueForce=off  SensingFrame=FollowerFrame  PositionTargetRotationMethod=None  PositionTargetRotationAngleUnits=deg  PositionTargetRotationStandardAxis=+Z  PositionTargetRotationAngle=0  PositionTargetRotationArbitraryAxis=[0 0 1]  PositionTargetFollAlignAxisA=+X  PositionTargetBaseAlignAxisA=+Y  PositionTargetFollAlignAxisB=+Y  PositionTargetBaseAlignAxisB=+Z  PositionTargetSpecify=off  PositionTargetPriority=High  VelocityTargetValue=[0 0 0]  VelocityTargetValueUnits=deg/s  VelocityTargetSpecify=off  VelocityTargetPriority=High  VelocityTargetInFollowerFrame=on  BlockFunction=simmechanics.library.joints.spherical_joint
  Tijelo_3_RIGID : Subsystem
  Tijelo_3_RIGID1 : Subsystem
  Tijelo_3_RIGID2 : Subsystem
  Tijelo_3_RIGID3 : Subsystem
  Tijelo_3_RIGID4 : Subsystem
  Tijelo_3_RIGID5 : Subsystem
  Transform3 : sm_lib/Frames and Transforms/Rigid Transform  TranslationMethod=StandardAxis  TranslationLengthUnit=mm  TranslationStandardAxis=-Z  TranslationStandardOffset=20  TranslationCartesianOffset=[80.000000000002558 4.2632564145606011e-14 -32.999999999999048]  TranslationROffset=0  TranslationROffsetUnits=m  TranslationZOffset=0  TranslationZOffsetUnits=m  TranslationThetaOffset=0  TranslationThetaOffsetUnits=deg  RotationMethod=None  RotationAngleUnits=rad  RotationStandardAxis=+Z  RotationAngle=0  RotationArbitraryAxis=[0 0 0]  FollAlignAxisA=+X  BaseAlignAxisA=+Y  FollAlignAxisB=+Y  BaseAlignAxisB=+Z  BlockFunction=simmechanics.library.frames_transforms.rigid_transform
  world_transf : PMIOPort  Port=1  Side=Left
  end_effector : PMIOPort  Port=2  Side=Right
  F1 : PMIOPort  Port=3  Side=Left
  F2 : PMIOPort  Port=4  Side=Left
  d1_s : PMIOPort  Port=5  Side=Right
  d2_s : PMIOPort  Port=6  Side=Right
  d3_s : PMIOPort  Port=7  Side=Right
  F3 : PMIOPort  Port=8  Side=Left
  end_effector1 : PMIOPort  Port=9  Side=Right
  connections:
  Postolje_donje_1_RIGID/RConn3 -- Revolute1/LConn1
  Koljeno_6_RIGID2/RConn1 -- Spherical/LConn1
  Koljeno_6_RIGID1/RConn1 -- Spherical1/LConn1
  G_ploca_2_RIGID/LConn2 -- Spherical1/RConn1
  G_ploca_2_RIGID/LConn1 -- Spherical2/RConn1
  G_ploca_2_RIGID/LConn3 -- Spherical/RConn1
  Revolute5/RConn1 -- Tijelo_3_RIGID/LConn1
  Koljeno_6_RIGID/RConn1 -- Spherical2/LConn1
  Postolje_donje_1_RIGID/RConn1 -- Revolute5/LConn1
  Tijelo_3_RIGID2/LConn1 -- Revolute1/RConn1
  Postolje_donje_1_RIGID/RConn2 -- Revolute3/LConn1
  d2_s/RConn1 -- Cylindrical1/RConn2
  d3_s/RConn1 -- Cylindrical/RConn2
  Cylindrical2/RConn1 -- Koljeno_6_RIGID/LConn1
  F3/RConn1 -- Cylindrical/LConn2
  d1_s/RConn1 -- Cylindrical2/RConn2
  Tijelo_3_RIGID1/LConn1 -- Revolute3/RConn1
  F1/RConn1 -- Cylindrical2/LConn2
  Koljeno_6_RIGID1/LConn1 -- Cylindrical1/RConn1
  F2/RConn1 -- Cylindrical1/LConn2
  Koljeno_6_RIGID2/LConn1 -- Cylindrical/RConn1
  world_transf/RConn1 -- Postolje_donje_1_RIGID/LConn1
  G_ploca_2_RIGID/RConn1 -- Transform3/LConn1 -- Postolje za vagu/LConn1
  Postolje za vagu/RConn1 -- end_effector/RConn1
  Tijelo_3_RIGID/RConn1 -- Tijelo_3_RIGID3/LConn1
  Tijelo_3_RIGID3/RConn1 -- Cylindrical2/LConn1
  Tijelo_3_RIGID1/RConn1 -- Tijelo_3_RIGID4/LConn1
  Tijelo_3_RIGID4/RConn1 -- Cylindrical1/LConn1
  Tijelo_3_RIGID2/RConn1 -- Tijelo_3_RIGID5/LConn1
  Tijelo_3_RIGID5/RConn1 -- Cylindrical/LConn1
  Transform3/RConn1 -- end_effector1/RConn1

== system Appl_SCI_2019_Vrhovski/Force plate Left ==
  Center of Presure : MATLAB Function  TreatAsAtomicUnit=on
  Donja ploca : Subsystem
  Gornja ploca : Subsystem
  Komponente senzora sile : Subsystem
  Senzori sile : Subsystem
  F : PMIOPort  Port=1  Side=Right
  B : PMIOPort  Port=2  Side=Left
  CoP_x : Outport
  CoP_y : Outport  Port=2
  Fz : Outport  Port=3
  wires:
  Komponente senzora sile/3(F1z) -> Center of Presure/1(Fz1)
  Komponente senzora sile/6(F2z) -> Center of Presure/2(Fz2)
  Komponente senzora sile/9(F3z) -> Center of Presure/3(Fz3)
  Komponente senzora sile/12(F4z) -> Center of Presure/4(Fz4)
  Center of Presure/1(CoP_x) -> CoP_x/1
  Center of Presure/2(CoP_y) -> CoP_y/1
  Center of Presure/3(F_suma) -> Fz/1
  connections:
  Senzori sile/RConn8 -- Komponente senzora sile/LConn4
  Senzori sile/RConn6 -- Komponente senzora sile/LConn3
  Komponente senzora sile/LConn2 -- Senzori sile/RConn4
  Senzori sile/RConn2 -- Komponente senzora sile/LConn1
  B/RConn1 -- Donja ploca/LConn1
  Gornja ploca/LConn3 -- Senzori sile/RConn5
  Senzori sile/RConn7 -- Gornja ploca/LConn4
  F/RConn1 -- Gornja ploca/RConn1
  Senzori sile/RConn3 -- Gornja ploca/LConn2
  Gornja ploca/LConn1 -- Senzori sile/RConn1
  Donja ploca/RConn4 -- Senzori sile/LConn4
  Donja ploca/RConn2 -- Senzori sile/LConn2
  Donja ploca/RConn3 -- Senzori sile/LConn3
  Donja ploca/RConn1 -- Senzori sile/LConn1
